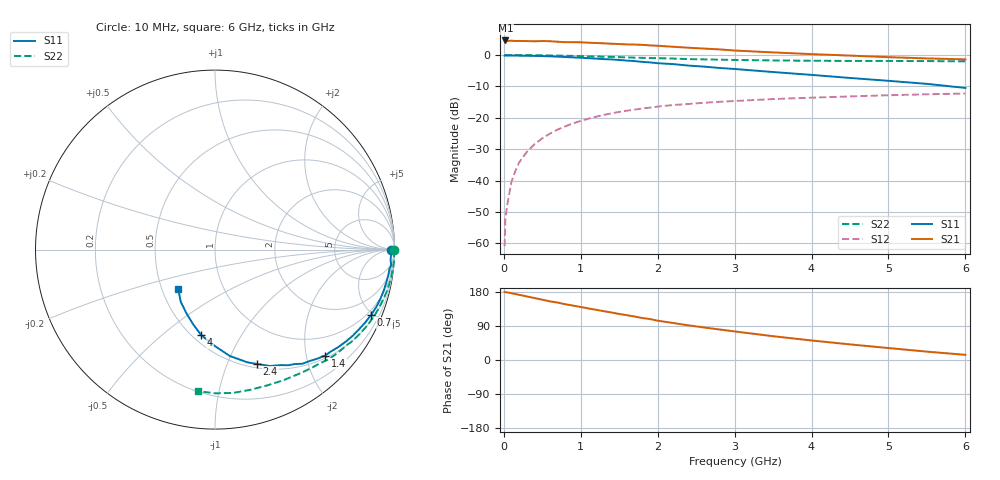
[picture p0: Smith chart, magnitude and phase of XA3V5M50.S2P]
! SIEMENS Discrete & RF Semiconductors
! BFY180
! Si NPN RF Bipolar Junction Transistor in MICRO-X
! VCE = 3.5 V  IC = 0.5 mA
! Common Emitter S-Parameters:  May  1997
# GHz  S  MA  R  50
!  f  S11  S21  S12  S22
! GHz  MAG  ANG  MAG  ANG  MAG  ANG  MAG  ANG
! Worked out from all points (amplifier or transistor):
!   36 points, 10 MHz to 6 GHz, reference 50 ohm
!   highest |S21| = 4.6 dB at 20 MHz (marker M1)
!   |S21| within 3 dB of that: start of sweep to 2.885 GHz
!   unconditionally stable (mu >= 1): 5.615 GHz to end of sweep
!   at 250 MHz: K = 0.06, MSG = 18.5 dB, |S12| = -32.5 dB
!   at 1.4 GHz: K = 0.39, MSG = 11.1 dB, |S12| = -18.6 dB
!   at 6 GHz: K = 1.02, MAG = 4.7 dB, |S12| = -12.3 dB
!   S11 on the Smith chart (normalised r, x): 10 MHz: 95, -16; 700 MHz: 0.74, -4.87; 1.4 GHz: 0.55, -2.37; 2.4 GHz: 0.54, -1.28; 4 GHz: 0.55, -0.69; 6 GHz: 0.61, -0.29
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0.01  0.9797 -0.2  1.683 179.8  0.0009 75.5  0.9978 -0.2
0.02  0.9835 -0.5  1.707 179.1  0.0025 83.5  0.9999 -0.4
0.05  0.9812 -1.7  1.669 178.1  0.0045 88.2  0.9989 -1.1
0.1  0.9801 -3.3  1.692 176.1  0.0097 87.7  0.9986 -2.4
0.2  0.9774 -6.5  1.678 171.9  0.0195 84.9  0.9978 -4.5
0.3  0.9733 -9.9  1.67 167.6  0.0287 83.0  0.9944 -6.8
0.4  0.9684 -13.2  1.656 163.5  0.0381 80.1  0.9939 -9.0
0.5  0.9618 -16.5  1.673 159.2  0.0471 77.4  0.9892 -11.3
0.6  0.9538 -19.6  1.66 154.7  0.0561 74.9  0.9853 -13.5
0.7  0.9428 -22.7  1.627 151.5  0.065 72.2  0.9797 -15.7
1  0.9052 -32.0  1.597 139.8  0.0894 65.0  0.9621 -22.2
1.1  0.8921 -34.9  1.572 136.1  0.0967 62.5  0.9553 -24.1
1.4  0.851 -43.9  1.513 125.4  0.1175 55.7  0.9327 -30.3
1.8  0.7773 -55.1  1.452 110.8  0.1407 48.3  0.9017 -37.4
2.2  0.7167 -64.8  1.355 97.7  0.1597 41.0  0.8783 -44.3
2.4  0.6789 -69.8  1.307 91.4  0.1658 38.0  0.8615 -47.4
2.8  0.6227 -78.1  1.23 80.6  0.1796 32.6  0.8431 -53.2
3.5  0.5359 -90.3  1.101 62.8  0.1988 24.5  0.8209 -62.7
4  0.4826 -99.2  1.034 51.5  0.2092 19.1  0.8102 -69.3
4.5  0.4311 -106.7  0.979 41.2  0.219 14.4  0.8055 -76.1
5.5  0.3473 -123.4  0.883 22.1  0.2369 5.2  0.8006 -90.0
6  0.2988 -133.3  0.853 13.6  0.2436 0.6  0.794 -96.9
